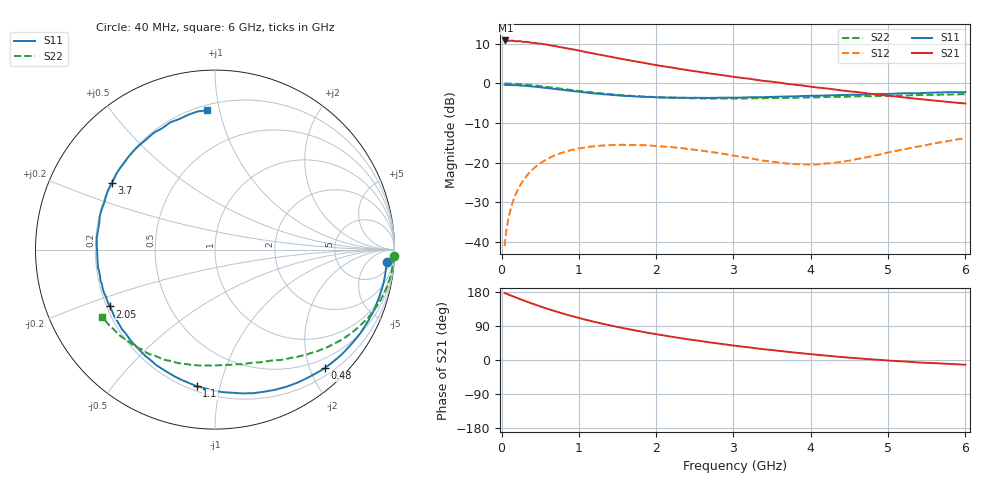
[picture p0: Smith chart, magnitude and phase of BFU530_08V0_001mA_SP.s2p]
! Filename:  P:\Prog\Test\Noise\ATS_data\Testdata_Net\03 Spar\BFU530_APG2013_40_A05_08p0V_001mA_SP_CM01_D.s2p
! Date/Time: Fri 26/Apr/2013 13:03:14
! BFU530_APG2013_40_A05_08p0V_1to25mA_SP_CM01_Bias1_R.s2p
! MDIF S-parameter v. bias file
! BFU530_APG2013_40_A05_08p0V_1to25mA_SP_CM01
! Date/time Wed Apr 24 16:58:28 2013
! bias mode 1
! bias variable = I_out
! VAR bias_var= 1
! VAR V_out= 8.0000
! VAR I_out= 1.0000
! VAR V_in= 0.7805
! VAR I_in= 0.0103
! Device data file deembeded for feedlines and parallel
! Original file: \03 Spar\BFU530_APG2013_40_A05_08p0V_001mA_SP_CM01_R.s2p
! Feed-files: PR047V01_250413_Feed1.s2p, PR047V01_250413_Feed2.s2p
! Parallel-file: PR047V01_250413_Par.s2p
# MHz S MA R 50
!  Freq-MHz  S11-mag  S11-arg  S21-mag  S21-arg  S12-mag  S12-arg  S22-mag  S22-arg
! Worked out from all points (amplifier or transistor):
!   98 points, 40 MHz to 6 GHz, reference 50 ohm
!   highest |S21| = 10.9 dB at 50 MHz (marker M1)
!   |S21| within 3 dB of that: start of sweep to 1.109 GHz
!   unconditionally stable (mu >= 1): 3.275 GHz to 4.946 GHz
!   at 300 MHz: K = 0.09, MSG = 17.2 dB, |S12| = -24.0 dB
!   at 1.6 GHz: K = 0.41, MSG = 10.8 dB, |S12| = -15.5 dB
!   at 6 GHz: K = 0.79, MSG = 4.4 dB, |S12| = -13.8 dB
!   S11 on the Smith chart (normalised r, x): 40 MHz: 12, -21; 480 MHz: 0.32, -2.25; 1.1 GHz: 0.23, -0.85; 2.05 GHz: 0.21, -0.24; 3.7 GHz: 0.20, +0.28; 6 GHz: 0.24, +0.92
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40  0.9608 -4.1  3.487 176.8  0.008792 86.9  0.9973 -2.0
50  0.9594 -5.0  3.492 175.8  0.01108 86.5  0.9993 -2.5
100  0.958 -10.0  3.453 171.9  0.02193 83.3  0.994 -5.3
140  0.9536 -14.2  3.463 168.6  0.03053 80.6  0.9907 -7.6
200  0.9492 -20.1  3.408 163.9  0.04322 76.6  0.9833 -10.8
320  0.9297 -32.1  3.355 154.6  0.06694 68.9  0.9641 -17.1
480  0.8998 -47.2  3.186 143.0  0.09469 59.4  0.9285 -24.7
600  0.8722 -58.2  3.084 134.8  0.112 52.9  0.8989 -30.0
700  0.8495 -66.9  2.957 128.3  0.1242 47.7  0.8741 -34.1
900  0.804 -82.9  2.716 116.5  0.144 38.7  0.828 -41.2
1050  0.7751 -94.1  2.542 108.2  0.1536 32.5  0.7929 -46.2
1100  0.7677 -97.6  2.481 105.7  0.156 30.6  0.783 -47.6
1300  0.733 -110.9  2.282 96.1  0.164 23.6  0.7482 -53.2
1500  0.7082 -123.2  2.088 87.2  0.1674 17.6  0.72 -58.3
1750  0.6826 -137.0  1.885 77.2  0.1666 11.1  0.6899 -64.1
2050  0.6669 -151.6  1.672 66.5  0.1603 4.9  0.6661 -70.7
2500  0.6593 -171.0  1.428 52.1  0.1453 -1.6  0.65 -79.9
3100  0.6626 166.6  1.177 35.7  0.118 -3.0  0.6463 -91.9
3700  0.6836 147.2  0.9859 21.6  0.09688 6.9  0.6577 -104.0
4100  0.7003 136.1  0.8845 13.5  0.09524 19.6  0.6682 -112.0
5200  0.7515 109.3  0.6664 -3.7  0.1469 40.1  0.7034 -133.8
6000  0.7764 93.2  0.5578 -12.4  0.204 38.0  0.7308 -149.2
